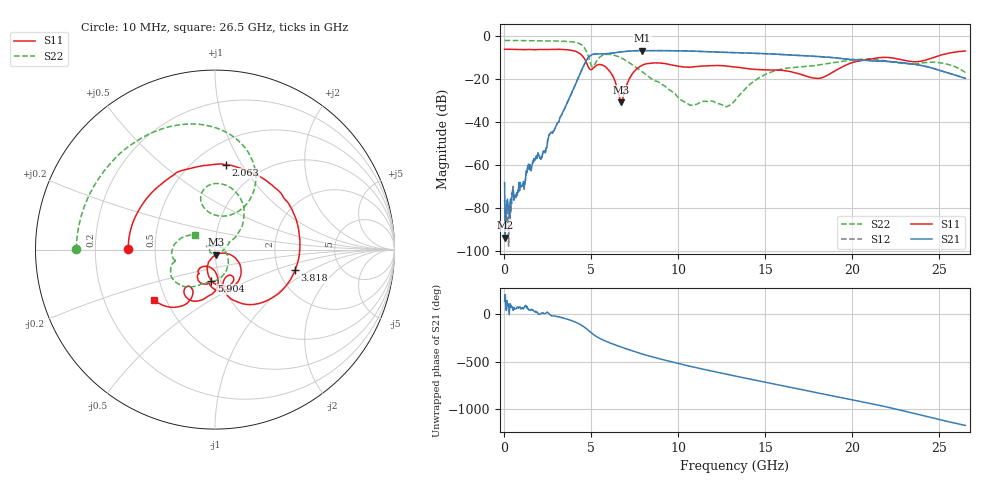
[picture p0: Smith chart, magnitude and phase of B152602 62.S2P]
!  2-Port S-parameters saved by WinCal
! VAR MeasName=S-Parameters (CALIBRATED_DATA) read from VNA (N5242A)
! VAR MeasDate=2016-1-5 16:34:37
! VAR NAME=B152602 62
! VAR FILENAME=B152602 62.S2P
! VAR DATE=2016-1-5 16:34:37
! VAR PHYS_PORTS=1,2
# Hz S DB R 50
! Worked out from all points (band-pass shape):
!   801 points, 10 MHz to 26.5 GHz, reference 50 ohm
!   highest |S21| = -6.94 dB at 7.924 GHz (marker M1); lowest = -93.7 dB at 43.11 MHz (marker M2)
!   |S21| within 3 dB of the highest: 4.851 GHz to 18.48 GHz (13.63 GHz wide, 117 % of centre)
!   lowest |S11| = -30.9 dB at 6.699 GHz (marker M3), VSWR 1.06, Z = 50.7 - j2.78 ohm
!   |S11| at or under -10 dB: 4.541 GHz to 24.73 GHz (20.19 GHz wide, 138 % of centre)
!   |S22| runs from -33.0 to -2.2 dB; largest |S21 - S12| = 0.0032
!   S11 on the Smith chart (normalised r, x): 10 MHz: 0.35, +0.00; 2.063 GHz: 0.70, +0.85; 3.818 GHz: 2.46, -0.72; 5.904 GHz: 0.91, -0.32; 26.5 GHz: 0.43, -0.30
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1e7  -6.32 179.5  -68.12 137.9  -76.18 37.2  -2.23 179.9
4.31125e7  -6.31 178.0  -93.65 -149.6  -83.93 80.6  -2.24 179.3
1.755625e8  -6.31 171.6  -75.86 97.0  -77.50 83.4  -2.24 177.3
1.0696e9  -6.52 130.3  -68.58 56.7  -68.45 52.3  -2.30 163.4
1.367612e9  -6.37 116.5  -59.95 61.8  -60.08 63.8  -2.33 158.7
2.062975e9  -6.44 82.8  -56.78 6.5  -56.68 6.2  -2.40 147.1
3.817938e9  -6.74 -14.4  -27.44 -61.8  -27.43 -61.8  -2.81 106.3
4.447075e9  -9.09 -60.3  -15.83 -115.0  -15.81 -114.9  -4.33 75.9
5.076212e9  -15.30 -57.6  -8.71 154.3  -8.70 154.4  -14.46 84.8
5.904025e9  -15.15 -96.5  -8.32 72.2  -8.31 72.2  -8.68 89.2
6.698725e9  -30.91 -74.5  -7.54 17.2  -7.54 17.2  -10.27 60.7
7.29475e9  -18.41 -21.9  -7.08 -20.5  -7.08 -20.5  -13.15 44.5
7.923888e9  -13.69 -47.0  -6.94 -57.0  -6.94 -56.9  -16.79 33.1
8.851038e9  -12.67 -78.8  -6.98 -104.0  -6.95 -104.0  -21.44 25.0
1.070534e10  -14.59 -99.4  -7.16 172.4  -7.14 172.4  -32.31 -82.3
1.3255e10  -14.58 -121.1  -7.88 71.3  -7.86 71.1  -30.09 35.1
1.527486e10  -15.88 -124.3  -8.47 -5.1  -8.46 -5.1  -17.04 -66.1
1.769208e10  -19.52 -118.0  -9.50 -95.3  -9.48 -95.2  -13.99 -109.2
1.971194e10  -13.34 -87.4  -10.91 -170.9  -10.88 -171.0  -11.57 -128.3
2.209604e10  -10.14 -120.6  -12.04 99.2  -11.97 98.8  -11.95 -161.1
2.401656e10  -11.73 -118.5  -13.89 15.3  -13.87 15.0  -12.61 -166.1
2.65e10  -7.12 -140.1  -19.76 -90.6  -19.75 -90.9  -17.14 144.3
